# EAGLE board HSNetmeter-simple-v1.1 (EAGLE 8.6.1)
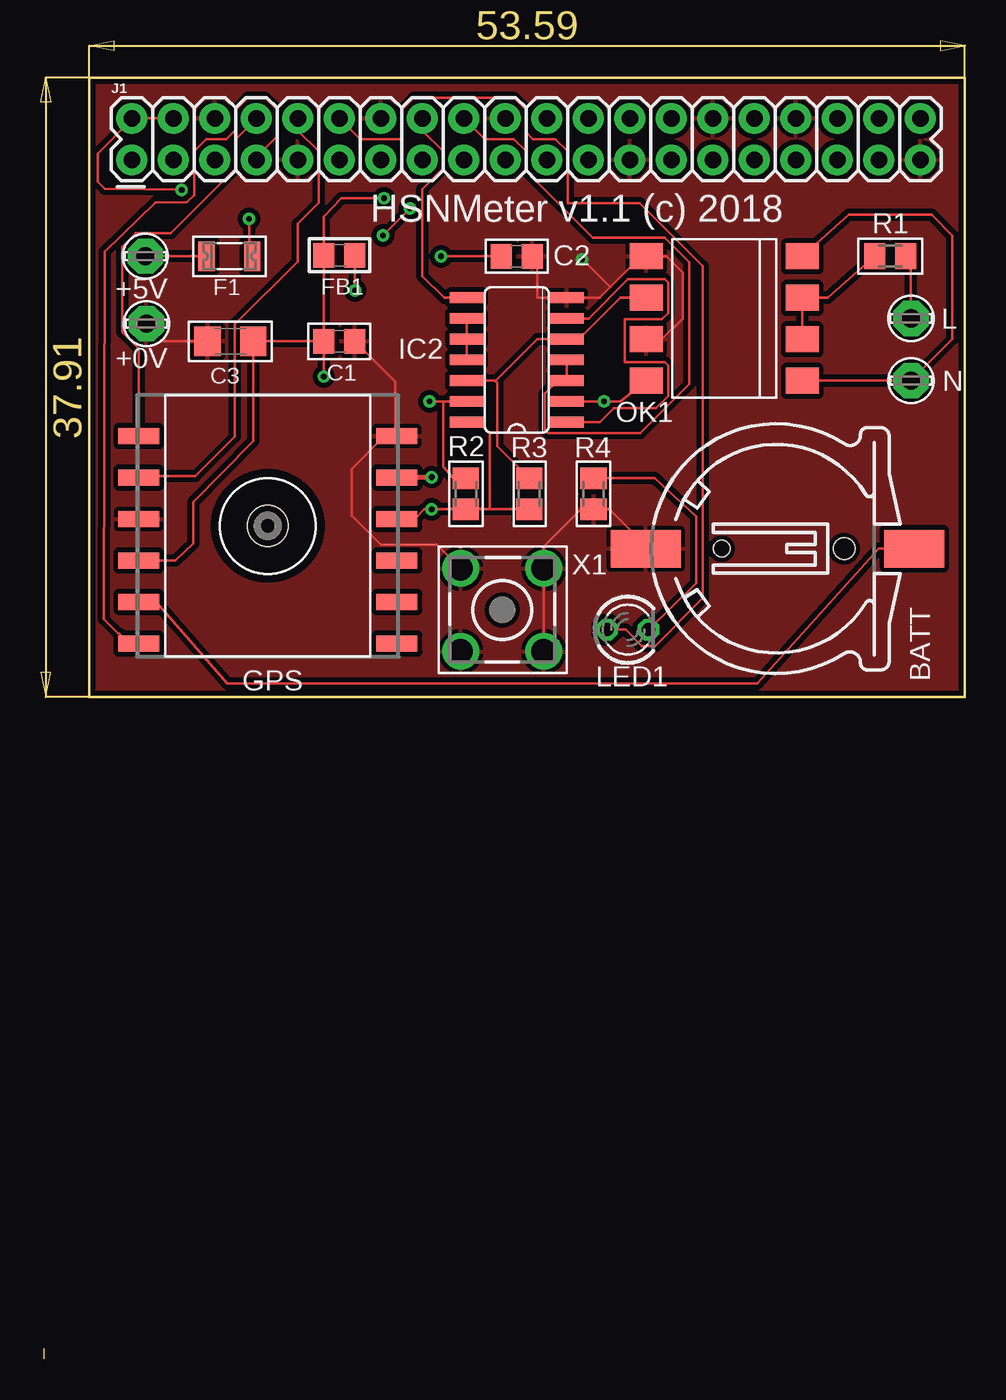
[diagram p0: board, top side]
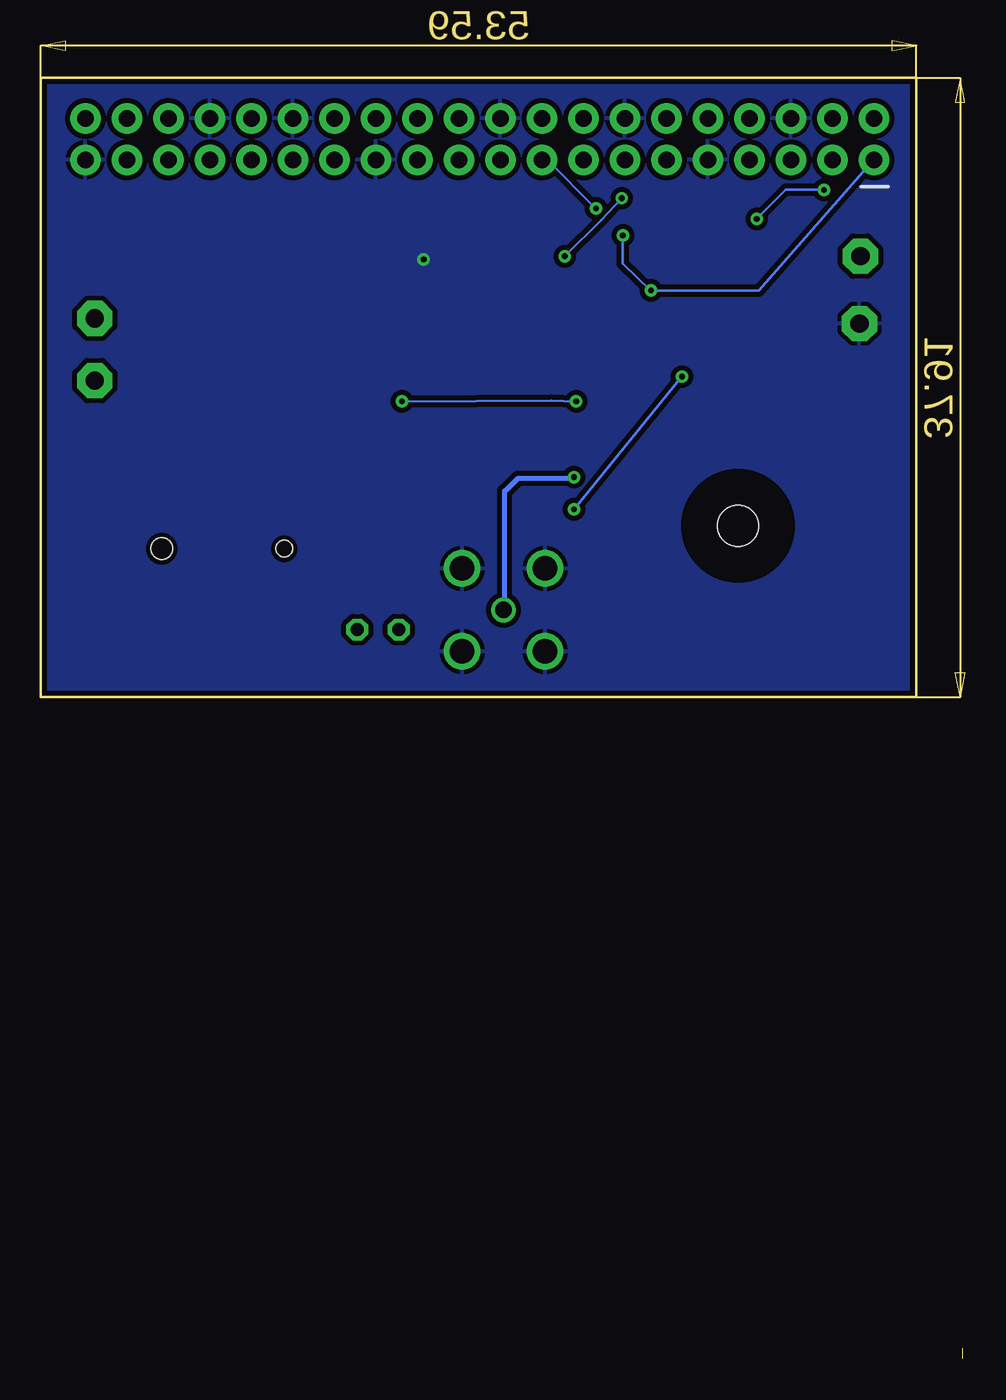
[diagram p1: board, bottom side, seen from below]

Size 56.56 x 80.69 mm. Coordinates in mm from the lower left corner, seen from the top.
Outline: 0.17,0.64 0.17,0
Outline: 2.97,78.42 56.56,78.42 56.56,40.51 2.97,40.51 2.97,78.42
Copper layers (1*16): Top 0.035mm / dielectric 1.5mm / Bottom 0.035mm
Design rules "default *": minimum track width 6mil, minimum drill 0.35mm, track to track 6mil, track to pad 6mil, pad to pad 6mil, via to via 6mil, smd to smd 6mil, copper to edge 12mil, drill to drill 6mil, minimum pad ring 10mil, minimum via ring 8mil, stop-mask expansion 4mil, vias tented up to drill 0mil, thermal gap 10mil
Net classes: 0 default: width 0.006 mm, clearance 0.254 mm
tKeepout: area 13.4,50.5 to 14.4,51.5
bKeepout: area 13.4,50.5 to 14.4,51.5

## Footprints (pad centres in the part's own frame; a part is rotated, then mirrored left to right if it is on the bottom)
LSP11 = drill 1.118 pad 2.159 octagon: MP 0,0
CH291-1220LF = smd 2.3 x 3.66: + 0,-2.296 | smd 2.3 x 4.3: - 0,14.146 | hole 1.3: 0,2 | hole 1: 0,9.5
C0805 = smd 1.3 x 1.5: 1 -0.95,0; 2 0.95,0
C1206 = smd 1.6 x 1.8: 1 -1.4,0; 2 1.4,0
1206L = smd 1 x 1.8: 1 -1.4,0; 2 1.4,0
0805 = smd 1.3 x 1.5: 1 -0.95,0; 2 0.95,0
QUECTEL_L80-M39 = smd 2.5 x 1: 1 7.9,-5.5; 2 7.9,-2.96; 3 7.9,-0.42; 4 7.9,2.12; 5 7.9,4.66; 6 7.9,7.2; 7 -7.9,7.2; 8 -7.9,4.66; 9 -7.9,2.12; 10 -7.9,-0.42; 11 -7.9,-2.96; 12 -7.9,-5.5
SO14 = smd 0.66 x 2.032: 1 -3.81,-3.073; 2 -2.54,-3.073; 3 -1.27,-3.073; 4 0,-3.073; 5 1.27,-3.073; 6 2.54,-3.073; 7 3.81,-3.073; 8 3.81,3.073; 9 2.54,3.073; 10 1.27,3.073; 11 0,3.073; 12 -1.27,3.073; 13 -2.54,3.073; 14 -3.81,3.073
2X20 = drill 1.016 pad 1.88: 1 0,0; 2 0,2.54; 3 2.54,0; 4 2.54,2.54; 5 5.08,0; 6 5.08,2.54; 7 7.62,0; 8 7.62,2.54; 9 10.16,0; 10 10.16,2.54; 11 12.7,0; 12 12.7,2.54; 13 15.24,0; 14 15.24,2.54; 15 17.78,0; 16 17.78,2.54; 17 20.32,0; 18 20.32,2.54; 19 22.86,0; 20 22.86,2.54; 21 25.4,0; 22 25.4,2.54; 23 27.94,0; 24 27.94,2.54; 25 30.48,0; 26 30.48,2.54; 27 33.02,0; 28 33.02,2.54; 29 35.56,0; 30 35.56,2.54; 31 38.1,0; 32 38.1,2.54; 33 40.64,0; 34 40.64,2.54; 35 43.18,0; 36 43.18,2.54; 37 45.72,0; 38 45.72,2.54; 39 48.26,0; 40 48.26,2.54
LED3MM = drill 0.813 octagon: A -1.27,0; K 1.27,0
DIL8-SMD = smd 1.6 x 2: 1 -3.81,-4.77; 2 -1.27,-4.77; 3 1.27,-4.77; 4 3.81,-4.77; 5 3.81,4.77; 6 1.27,4.77; 7 -1.27,4.77; 8 -3.81,4.77
M0805 = smd 1.3 x 1.6: 1 -0.95,0; 2 0.95,0
DRIL-2,5 = hole 2.5: 0,0
BU-SMC-V = drill 1.016: 1 0,0 | drill 1.5: 2 -2.54,2.54; 3 2.54,2.54; 4 2.54,-2.54; 5 -2.54,-2.54

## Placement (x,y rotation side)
+0V  LSP11  [LSP11]  6.46,63.37 0 top
+5V  LSP11  [LSP11]  6.4,67.5 0 top
BATT  CH291-1220LF  [CH291-1220LF]  51.16,49.59 90 top
C1  100nF  [C0805]  18.27,62.29 0 top
C2  100nF  [C0805]  29.13,67.5 0 top
C3  10uF  [C1206]  11.6,62.29 180 top
F1  1206L110TH  [1206L]  11.54,67.5 0 top
FB1  Ferrite  [0805]  18.27,67.56 0 top
GPS  L80-M39  [QUECTEL_L80-M39]  13.89,50.99 180 top
IC2  74HC132D  [SO14]  29.13,61.15 90 top
J1  RASPBERRYPI-40-PIN-GPIO_PTH_NO_SHROUD  [2X20]  5.57,73.41 0 top
L  LSP11  [LSP11]  53.26,63.69 0 top
LED1  GN  [LED3MM]  35.92,44.64 0 top
N  LSP11  [LSP11]  53.26,59.88 0 top
OK1  LTV826S  [DIL8-SMD]  41.83,63.69 90 top
R1  330 Ohm  [M0805]  51.99,67.5 180 top
R2  10kOhm  [M0805]  26.02,52.96 90 top
R3  10kOhm  [M0805]  29.89,52.96 270 top
R4  330 Ohm  [M0805]  33.83,52.96 90 top
U$2  [DRIL-2,5]  13.89,50.99 0 top
X1  BU-SMC-V  [BU-SMC-V]  28.24,45.85 0 top

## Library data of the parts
+0V +5V L N = solpad
BATT = battery
C1-C3 R1-R4 = resistor
F1 = polyfuse-smd_10; MF: Littelfuse; MPN: 1206L110TH; OC_FARNELL: 2383294; OC_NEWARK: 64R8194
FB1 = microbuilder
GPS = L80-M39; AVAILABILITY: Bad; DESCRIPTION: GPS Receiver 1575.42MHz 3.3V 12-Pin; MF: Quectel; MP: L80-M39; PACKAGE: None; PRICE: 8.97 USD
IC2 = 74xx-eu
J1 = SparkFun-Connectors
LED1 = led
OK1 = optocoupler; OC_FARNELL: unknown; OC_NEWARK: unknown
U$2 = special
X1 = con-coax; OC_FARNELL: unknown; OC_NEWARK: unknown

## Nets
3.3V: FB1.2 J1.1 J1.17
5V: F1.2 J1.2 J1.4
50HZ: IC2.3 IC2.4 J1.18
100HZ: IC2.8 J1.16
GND: +0V.MP BATT.- C1.2 C2.2 C3.2 GPS.3 GPS.12 IC2.7 J1.6 J1.9 J1.14 J1.20 J1.25 J1.30 J1.34 J1.39 OK1.5 OK1.7 R4.1 X1.2 X1.3 X1.4 X1.5
LED: J1.12 LED1.A
N$2: L.MP R1.1
N$3: LED1.K R4.2
N$4: N.MP OK1.1 OK1.4
N$6: +5V.MP F1.1
N$8: GPS.6 J1.7
N$9: OK1.2 OK1.3 R1.2
N$10: GPS.1 J1.8
N$11: GPS.2 J1.10
N$12: IC2.2 IC2.13 OK1.8 R2.2
N$13: IC2.5 IC2.12 OK1.6 R3.1
N$15: IC2.1 IC2.6
N$16: IC2.9 IC2.10 IC2.11
N$17: GPS.11 X1.1
N$18: BATT.+ GPS.5
VCC: C1.1 C2.1 C3.1 FB1.1 GPS.4 GPS.10 IC2.14 R2.1 R3.2

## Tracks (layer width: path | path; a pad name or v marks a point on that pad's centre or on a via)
3.3V  (via drill 0.35)
  Top 0.152: v19.22,65.41 FB1.2 | v22.59,70.42 v20.94,68.77
  Bottom 0.152: J1.1 12.62,65.41 v19.22,65.41 20.94,67.06 v20.94,68.77 | v22.59,70.42 25.57,73.41 J1.17
5V  (via drill 0.35)
  Top 0.152: J1.4 J1.2 5.57,75.88 3.47,73.79 3.47,72.07 3.92,71.63 v8.62,71.56 | v12.75,69.79 12.75,68.45 12.94,68.26 F1.2
  Bottom 0.152: v12.75,69.79 10.97,71.56 10.71,71.56 v8.62,71.56
50HZ
  Top 0.152: IC2.4 IC2.3 31.66,59.88 30.86,59.08 30.86,56.87 31.05,56.68 36.7,56.68 39.7,59.68 39.7,67.13 38.2,68.63 33.78,68.63 29.7,72.71 29.7,73.93 28.96,74.68 27.16,74.68 J1.18
100HZ
  Top 0.152: J1.16 23.35,75.2 24.62,73.93 24.62,72.88 23.35,71.61 23.35,66.29 24.68,64.96 IC2.8
GND  (via drill 0.35)
  Top 0.152: 34.84,65.6 34.21,64.96 IC2.7 30.4,64.96 30.4,67.5 C2.2 | 34.84,65.6 36.75,67.5 OK1.5 38.27,67.5 39.29,66.48 39.29,63.69 38.02,62.42 OK1.7 | GPS.3 5.99,50.99 5,50.99 | C3.2 7.54,62.29 | BATT.- 37.19,49.59 34.78,52.01 R4.1 33.76,52.01 33.07,52.01 30.78,49.72 X1.3 X1.4 | 21.7,56.52 21.76,56.52 GPS.12 | 21.7,56.52 21.06,56.52 19.03,54.48 19.03,51.63 20.81,49.85 24.24,49.85 X1.2 | C1.2 21.7,59.81 21.7,56.52 | 34.84,65.6 v33.13,67.31
  pour Top (isolate 0.305): 2.97,78.42 56.56,78.42 56.56,40.51 2.97,40.51
  pour Bottom (isolate 0.305): 2.97,78.42 56.56,78.42 56.56,40.51 2.97,40.51
LED
  Top 0.152: J1.12 19.54,74.68 22.08,74.68 22.08,76.47 22.82,77.22 28.96,77.22 29.7,76.47 29.7,75.08 30.11,74.68 31.5,74.68 32.24,73.93 32.24,70.74 36.66,70.74 40.52,66.88 40.52,51.57 40.53,51.41 40.52,51.4 40.52,46.57 37.6,43.65 36.78,43.65 35.79,44.64 LED1.A
N$2
  Top 0.152: L.MP 53.26,67.5 R1.1
N$3
  Top 0.152: R4.2 37.57,53.91 40.11,51.56 40.11,47.5 LED1.K
N$4
  Top 0.152: OK1.1 N.MP 55.8,62.42 55.8,68.77 54.53,70.04 49.45,70.04 OK1.4
N$6
  Top 0.152: +5V.MP F1.1
N$8
  Top 0.152: J1.7 13.19,73.58 14.46,74.85 14.46,76.47 13.72,77.22 12.66,77.22 11.92,76.47 11.92,75.25 11.35,74.68 10.12,74.68 9.38,73.93 9.38,71.23 8.94,70.8 6.99,70.79 3.92,67.78 3.86,45.28 4.74,44.39 4.81,44.39 5.4,43.79 GPS.6
N$9
  Top 0.152: OK1.2 OK1.3 48.18,64.96 R1.2
N$10
  Top 0.152: J1.8 11.92,74.68 11.92,72.88 7.95,68.91 5.81,68.91 4.99,68.08 4.99,62.85 5.99,61.85 GPS.1
N$11
  Top 0.152: J1.10 15.73,75.2 17,73.93 17,70.79 15.72,69.51 15.72,67.18 11.87,63.33 11.87,56.47 9.44,54.04 6.08,54.04 GPS.2
N$12  (via drill 0.35)
  Top 0.152: OK1.8 35.48,58.61 v34.46,58.61 IC2.2 | 24.62,58.61 24.62,54.61 25.26,53.91 R2.2 | 24.62,58.61 v23.8,58.61 | 24.62,58.61 IC2.13
  Bottom 0.152: v34.46,58.61 25.32,58.67 v23.8,58.61
N$13
  Top 0.152: OK1.6 35.48,64.96 32.94,62.42 IC2.5 30.4,62.42 27.86,59.88 | 27.86,59.88 IC2.12 | R3.1 27.92,55.88 27.92,59.75 27.86,59.82 27.86,59.88
N$15
  Top 0.152: IC2.6 33.52,63.69 35.92,66.09 38.2,66.09 38.39,65.9 38.39,64.02 38,63.64 35.73,63.64 35.73,61.01 38.2,61.01 38.39,60.82 38.39,58.94 37.63,58.19 35.06,58.19 34.21,57.34 32.94,57.34 IC2.1
N$16
  Top 0.152: IC2.9 IC2.10 IC2.11
N$17  (via drill 0.35)
  Top 0.305: v23.92,53.98 21.83,53.98 GPS.11
  Bottom 0.305: X1.1 28.18,45.91 28.18,53.15 28.05,53.21 27.35,53.91 23.92,53.91 23.8,53.98 v23.92,53.98
N$18
  Top 0.152: 5,45.91 GPS.5 6.01,46.35 7.03,46.35 11.41,41.34 43.86,41.34 51.29,49.59 BATT.+
VCC  (via drill 0.35)
  Top 0.152: C1.1 C3.1 13,56.2 9.32,52.45 9.32,49.91 8.21,48.87 GPS.4 | 27.48,52.01 R3.2 | 27.48,52.01 26.08,52.01 R2.1 25.95,52.01 v23.92,52.01 23.48,52.01 22.91,51.44 21.83,51.44 GPS.10 | 27.48,52.01 27.48,56.64 26.78,57.34 IC2.14 | C1.1 17.32,62.36 17.32,67.5 FB1.1 17.32,67.63 17.32,69.91 18.4,71.06 v21,71.06 | v17.32,60.13 17.32,62.23 C1.1 | v24.49,67.5 28.11,67.5 28.18,67.44 28.24,67.5 C2.1
  Bottom 0.152: v23.92,52.01 v17.32,60.13 | v21,71.06 22.27,69.72 v24.49,67.5

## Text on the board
tPlace: HSNMeter v1.1 (c) 2018

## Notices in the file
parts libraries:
microbuilder: This work is placed in the public domain, and may be freely used for commercial and non-commercial work with the following conditions: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
SparkFun-Connectors: Licensing: Creative Commons ShareAlike 4.0 International - https://creativecommons.org/licenses/by-sa/4.0
